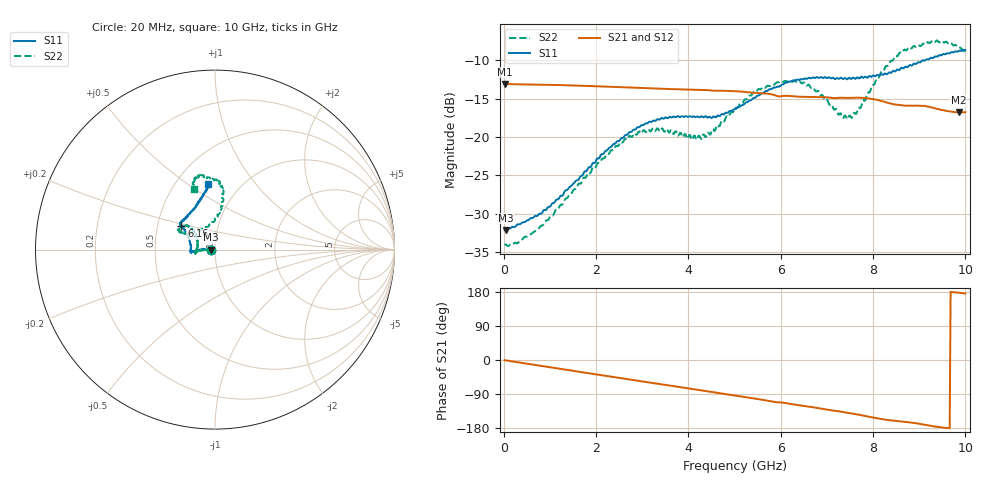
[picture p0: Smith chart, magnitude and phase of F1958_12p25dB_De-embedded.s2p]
! Integrated Device Technology
! Corporate Headquarters
! 6024 Silver Creek Valley Road
! San Jose, CA 95138  USA
! Phone:  1-408-284-8200
! Toll Free:  1-800-223-1366
! Webpage:  http://www.idt.com/
! Timing and RF Division
! 515 Groton Road, Suite 102
! Westford, MA 01886-6024
! Device:  F1958
! Description: 7-bit 0.25 dB Digital Step Attenuator
! Frequency:  0.001 -  6.000 GHz
! Package:  4x4 mm Thin QFN Plastic Package: 24 pin
! Ports:  2 RF, 12 DC
!  Pin  1  = D0
!  Pin  2  = VDD
!  Pin  3  = VMODE
!  Pin  4  = GND
!  Pin  5  = RF1  =  Port 1
!  Pin  6  = GND
!  Pin  7  = GND
!  Pin  8  = GND
!  Pin  9  = GND
!  Pin 10  = GND
!  Pin 11  = GND
!  Pin 12  = GND
!  Pin 13  = GND
!  Pin 14  = RF2  =  Port 2
!  Pin 15  = GND
!  Pin 16  = LE
!  Pin 17  = CLK
!  Pin 18  = DATA
!  Pin 19  = D6
!  Pin 20  = D5
!  Pin 21  = D4
!  Pin 22  = D3
!  Pin 23  = D2
!  Pin 24  = D1
! State:  49
! Atten State:  12.25 dB
! Voltage:  +3.30 Volts
! Current:  0.257 mA
! Data:  The device was measured on a F1958 evaluation board which has
!  individual transmission lines to the RF pins.  Data was collected
!  using a calibrated network analyzer.  The evaluation board was
!  de-embedded using Automatic Fixture Removal (AFR).
!  The reference plane is the edge of the package pin.
! Misc:
!  Action Tracker AT0419
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# GHz S dB R 50
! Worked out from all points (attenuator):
!   500 points, 20 MHz to 10 GHz, reference 50 ohm
!   highest |S21| = -13.09 dB at 20 MHz (marker M1); lowest = -16.8 dB at 9.86 GHz (marker M2)
!   lowest |S11| = -32.1 dB at 40 MHz (marker M3), VSWR 1.05, Z = 47.6 - j0.0871 ohm
!   |S11| at or under -10 dB: start of sweep to 9.132 GHz
!   |S22| runs from -34.2 to -7.4 dB; largest |S21 - S12| = 0.00067
!   S11 on the Smith chart (normalised r, x): 20 MHz: 0.95, -0.00; 6.16 GHz: 0.66, +0.18; 10 GHz: 0.71, +0.60
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0.02  -32.09 -177.9  -13.09 -0.5  -13.09 -0.5  -34.05 -177.7
0.04  -32.10 -177.9  -13.10 -0.9  -13.10 -0.9  -33.97 -176.7
0.32  -31.36 178.4  -13.15 -6.3  -13.15 -6.3  -33.72 179.4
0.72  -30.28 178.9  -13.19 -13.8  -13.18 -13.8  -32.07 -179.0
1.7  -25.02 179.6  -13.34 -32.3  -13.33 -32.2  -25.66 -178.5
2.6  -20.02 -177.5  -13.54 -49.0  -13.52 -49.0  -20.50 -174.9
2.92  -18.72 -175.2  -13.60 -55.0  -13.59 -55.1  -19.31 -172.2
3.36  -17.73 -173.6  -13.72 -63.2  -13.72 -63.3  -19.13 -168.7
4.26  -17.38 179.4  -13.87 -79.6  -13.89 -79.6  -20.14 168.0
4.52  -17.46 173.4  -13.97 -84.6  -13.98 -84.6  -18.97 153.8
5.02  -16.38 159.7  -14.05 -93.8  -14.06 -93.8  -16.20 139.3
5.54  -14.56 149.3  -14.29 -103.8  -14.29 -103.8  -13.79 140.1
6.16  -12.85 145.2  -14.64 -114.9  -14.66 -114.8  -12.82 148.8
6.68  -12.29 142.4  -14.80 -124.3  -14.81 -124.2  -13.61 152.3
7.3  -12.29 136.1  -14.90 -136.2  -14.91 -136.0  -16.92 130.1
7.5  -12.35 133.3  -14.92 -140.1  -14.92 -140.0  -17.21 111.9
7.68  -12.32 130.3  -14.89 -144.0  -14.88 -144.0  -16.21 95.5
8.34  -11.62 114.7  -15.59 -158.7  -15.59 -158.8  -10.59 80.8
8.68  -10.97 107.8  -15.92 -163.1  -15.91 -163.0  -8.61 85.5
9.26  -9.69 100.0  -16.15 -174.1  -16.16 -174.1  -7.60 98.6
9.86  -8.80 95.9  -16.81 177.5  -16.84 177.6  -8.39 108.0
10  -8.70 96.0  -16.78 175.4  -16.80 175.5  -8.94 108.9
